ORGANIZATION_BLOCK "Hardware Interrupt 5"
TITLE =
VERSION : 0.1


VAR_TEMP
  OB45_EV_CLASS : BYTE ;	//Bits 0-3 = 1 (Coming event), Bits 4-7 = 1 (Event class 1)
  OB45_STRT_INF : BYTE ;	//16#41/42/43/44 (Interrupt 1/2/3/4)
  OB45_PRIORITY : BYTE ;	//21 (Priority of 1 is lowest)
  OB45_OB_NUMBR : BYTE ;	//45 (Organization block 45, OB45)
  OB45_RESERVED_1 : BYTE ;	//Reserved for system
  OB45_RESERVED_2 : BYTE ;	//Reserved for system
  OB45_MDL_ADDR : WORD ;	//Base address of module initiating interrupt
  OB45_POINT_ADDR : DWORD ;	//Address of interrupt point on module
  OB45_DATE_TIME : DATE_AND_TIME ;	//Date and time OB45 started
END_VAR
BEGIN
END_ORGANIZATION_BLOCK

